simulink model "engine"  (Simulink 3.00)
settings: Solver=ode45  SolverMode=SingleTasking  StartTime=0.0  StopTime=10  RelTol=1e-3  AbsTol=1e-6

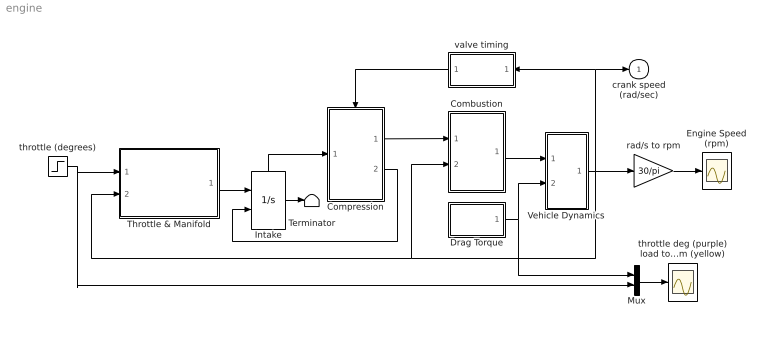
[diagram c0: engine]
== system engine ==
  Combustion : Subsystem
  Compression : Subsystem
  Drag Torque : Subsystem
  Engine Speed (rpm) : Scope
  Intake : Integrator  ExternalReset=either  InitialConditionSource=internal  InitialCondition=0  LimitOutput=off  UpperSaturationLimit=inf  LowerSaturationLimit=-inf  ShowSaturationPort=off  ShowStatePort=on  AbsoluteTolerance=auto
  Mux : Mux  Inputs=2
  Terminator : Terminator
  Throttle & Manifold : Subsystem
  Vehicle Dynamics : Subsystem
  rad/s to rpm : Gain  Gain=30/pi  SaturateOnIntegerOverflow=on
  throttle (degrees) : Step  Time=5  Before=8.973  After=11.93  SampleTime=0
  throttle deg (purple) load torque Nm (yellow) : Scope
  valve timing : Subsystem  Orientation=left
  crank speed (rad/sec) : Outport  Port=1  InitialOutput=0
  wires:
  valve timing/1(edge180) -> Compression/Trigger
  Intake/State -> Compression/1(mass(k+1))
  Intake/1 -> Terminator/1
  Throttle & Manifold/1(Mass Airflow Rate) -> Intake/1
  throttle (degrees)/1 -> Mux/2, Throttle & Manifold/1(Throttle Ang.)
  Compression/2(trigger) -> Intake/2
  Vehicle Dynamics/1(N) -> rad/s to rpm/1, crank speed (rad/sec)/1, valve timing/1(N), Combustion/2(N), Throttle & Manifold/2("Engine Speed, N")
  Compression/1(mass(k)) -> Combustion/1(Air Charge)
  rad/s to rpm/1 -> Engine Speed (rpm)/1
  Combustion/1(Torque) -> Vehicle Dynamics/1(Teng)
  Mux/1 -> throttle deg (purple) load torque Nm (yellow)/1
  Drag Torque/1(Load) -> Vehicle Dynamics/2(Tload), Mux/1

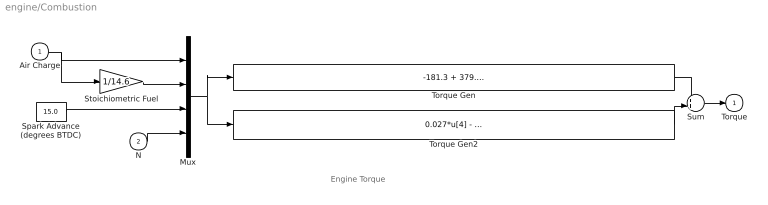
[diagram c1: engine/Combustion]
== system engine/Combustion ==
  note: Engine Torque
  Air Charge : Inport  Port=1  PortWidth=-1  SampleTime=-1  DataType=auto
  N : Inport  Port=2  PortWidth=-1  SampleTime=-1  DataType=auto
  Mux : Mux  Inputs=4
  Spark Advance (degrees BTDC) : Constant  Value=15.0
  Stoichiometric Fuel : Gain  Gain=1/14.6  SaturateOnIntegerOverflow=on
  Sum : Sum  Inputs=++  SaturateOnIntegerOverflow=on
  Torque Gen : Fcn  Expr=-181.3 + 379.36*u[1] + 21.91*u[1]/u[2] - (0.85*u[1]*u[1])/(u[2]*u[2]) + 0.26*u[3] - 0.0028*u[3]*u[3]
  Torque Gen2 : Fcn  Expr=0.027*u[4] - 0.000107*u[4]*u[4] + 0.00048*u[4]*u[3] + 2.55*u[3]*u[1] - 0.05*u[3]*u[3]*u[1]
  Torque : Outport  Port=1  InitialOutput=0
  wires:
  Sum/1 -> Torque/1
  Torque Gen/1 -> Sum/1
  Torque Gen2/1 -> Sum/2
  Mux/1 -> Torque Gen2/1, Torque Gen/1
  Air Charge/1 -> Mux/1, Stoichiometric Fuel/1
  N/1 -> Mux/4
  Spark Advance (degrees BTDC)/1 -> Mux/3
  Stoichiometric Fuel/1 -> Mux/2

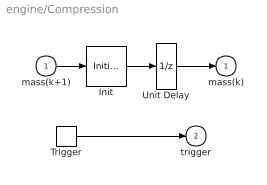
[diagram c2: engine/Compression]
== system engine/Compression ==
  mass(k+1) : Inport  Port=1  PortWidth=-1  SampleTime=-1  DataType=auto
  Trigger : TriggerPort  TriggerType=either  ShowOutputPort=on  OutputDataType=auto
  Init : InitialCondition  Value=0.152
  Unit Delay : UnitDelay  X0=0.152  SampleTime=-1
  mass(k) : Outport  Port=1  InitialOutput=0.152
  trigger : Outport  Port=2  InitialOutput=-1
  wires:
  Trigger/1 -> trigger/1
  Unit Delay/1 -> mass(k)/1
  mass(k+1)/1 -> Init/1
  Init/1 -> Unit Delay/1

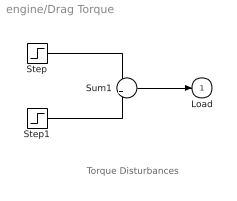
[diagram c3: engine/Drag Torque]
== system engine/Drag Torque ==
  note: Torque Disturbances
  Step : Step  Time=2  Before=25  After=20  SampleTime=0
  Step1 : Step  Time=8  Before=0  After=5  SampleTime=0
  Sum1 : Sum  Inputs=++  SaturateOnIntegerOverflow=on
  Load : Outport  Port=1  InitialOutput=0
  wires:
  Sum1/1 -> Load/1
  Step/1 -> Sum1/1
  Step1/1 -> Sum1/2

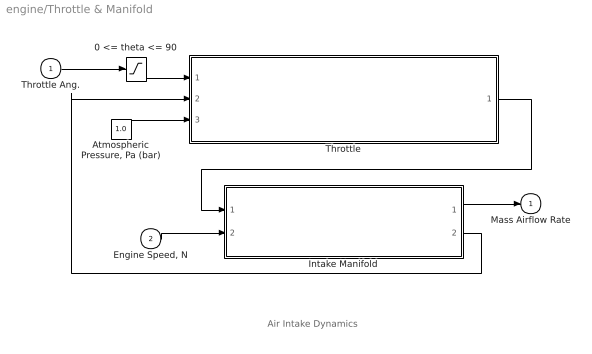
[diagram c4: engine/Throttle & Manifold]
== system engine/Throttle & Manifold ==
  note: Air Intake Dynamics
  Throttle Ang. : Inport  Port=1  PortWidth=-1  SampleTime=-1  DataType=auto
  "Engine Speed, N" : Inport  Port=2  PortWidth=-1  SampleTime=-1  DataType=auto
  0 <= theta <= 90 : Saturate  UpperLimit=90  LowerLimit=0
  "Atmospheric Pressure, Pa (bar)" : Constant  Value=1.0
  Intake Manifold : Subsystem
  Throttle : Subsystem
  Mass Airflow Rate : Outport  Port=1  InitialOutput=0
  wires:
  0 <= theta <= 90/1 -> Throttle/1("Throttle Angle, theta (deg)")
  Throttle Ang./1 -> 0 <= theta <= 90/1
  Throttle/1("Throttle  Flow, mdot  (g/s)") -> Intake Manifold/1(mdot Input  (g/s))
  "Engine Speed, N"/1 -> Intake Manifold/2(N (rad/sec))
  Intake Manifold/2("Manifold Pressure, Pm (bar)") -> Throttle/2("Manifold Pressure, Pm (bar)")
  Intake Manifold/1(mdot to  Cylinder  (g/s)) -> Mass Airflow Rate/1
  "Atmospheric Pressure, Pa (bar)"/1 -> Throttle/3("Atmospheric Pressure, Pa (bar) ")

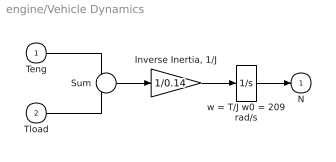
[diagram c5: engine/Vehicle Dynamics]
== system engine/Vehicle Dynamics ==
  Teng : Inport  Port=1  PortWidth=-1  SampleTime=-1  DataType=auto
  Tload : Inport  Port=2  PortWidth=-1  SampleTime=-1  DataType=auto
  "Inverse Inertia, 1/J" : Gain  Gain=1/0.14  SaturateOnIntegerOverflow=on
  Sum : Sum  Inputs=+-  SaturateOnIntegerOverflow=on
  w = T/J w0 = 209 rad/s : Integrator  ExternalReset=none  InitialConditionSource=internal  InitialCondition=209.48  LimitOutput=off  UpperSaturationLimit=inf  LowerSaturationLimit=-inf  ShowSaturationPort=off  ShowStatePort=off  AbsoluteTolerance=auto
  N : Outport  Port=1  InitialOutput=0
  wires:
  Tload/1 -> Sum/2
  Teng/1 -> Sum/1
  Sum/1 -> "Inverse Inertia, 1/J"/1
  w = T/J w0 = 209 rad/s/1 -> N/1
  "Inverse Inertia, 1/J"/1 -> w = T/J w0 = 209 rad/s/1

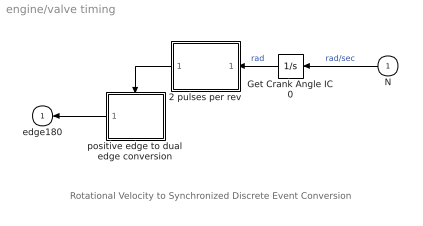
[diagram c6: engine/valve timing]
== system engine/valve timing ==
  note: Rotational Velocity to Synchronized Discrete Event Conversion
  N : Inport  Orientation=left  Port=1  PortWidth=-1  SampleTime=-1  DataType=auto
  2 pulses per rev : Subsystem  Orientation=left  mask(synchronous rotational pulse generator){Nper=2}
      mask prompts: Nper "pulses per rev (Nper)"
      mask help: A continuous angular position input (radians) is used to generate Nper timing pulses each revolution. When using a variable step-size solver, the pulses are issued at the precise instants the input crosses 2*pi/Nper. In addition, the solver is prevented from taking any steps that are so large that an entire pulse is missed.
      mask init:
      | delta = 2*pi/Nper;
  Get Crank Angle IC 0 : Integrator  Orientation=left  ExternalReset=none  InitialConditionSource=internal  InitialCondition=0  LimitOutput=off  UpperSaturationLimit=inf  LowerSaturationLimit=-inf  ShowSaturationPort=off  ShowStatePort=off  AbsoluteTolerance=auto
  positive edge to dual edge conversion : Subsystem  Orientation=left
  edge180 : Outport  Orientation=left  Port=1  InitialOutput=-1
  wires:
  N/1 -> Get Crank Angle IC 0/1  "rad/sec"
  Get Crank Angle IC 0/1 -> 2 pulses per rev/1(theta)  "rad"
  positive edge to dual edge conversion/1(trigger) -> edge180/1
  2 pulses per rev/1(trigger) -> positive edge to dual edge conversion/Trigger

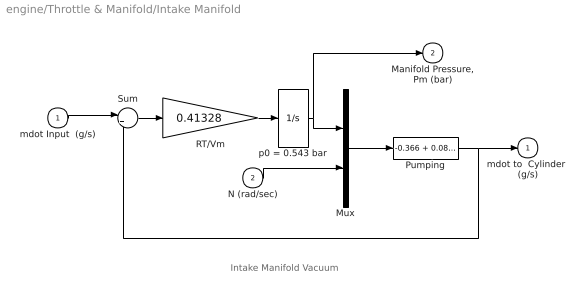
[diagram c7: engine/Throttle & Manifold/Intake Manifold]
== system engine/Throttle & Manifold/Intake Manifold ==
  note: Intake Manifold Vacuum
  mdot Input  (g/s) : Inport  Port=1  PortWidth=-1  SampleTime=-1  DataType=auto
  N (rad/sec) : Inport  Port=2  PortWidth=-1  SampleTime=-1  DataType=auto
  Mux : Mux  Inputs=2
  Pumping : Fcn  Expr=-0.366 + 0.08979*u[1]*u[2] - 0.0337*u[2]*u[1]*u[1] + 0.0001*u[1]*u[2]*u[2]
  RT/Vm : Gain  Gain=0.41328  SaturateOnIntegerOverflow=on
  Sum : Sum  Inputs=|+-  SaturateOnIntegerOverflow=on
  p0 = 0.543 bar : Integrator  ExternalReset=none  InitialConditionSource=internal  InitialCondition=.543  LimitOutput=off  UpperSaturationLimit=inf  LowerSaturationLimit=-inf  ShowSaturationPort=off  ShowStatePort=off  AbsoluteTolerance=auto
  mdot to  Cylinder  (g/s) : Outport  Port=1  InitialOutput=0
  "Manifold Pressure, Pm (bar)" : Outport  Port=2  InitialOutput=0
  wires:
  mdot Input  (g/s)/1 -> Sum/1
  RT/Vm/1 -> p0 = 0.543 bar/1
  N (rad/sec)/1 -> Mux/2
  Mux/1 -> Pumping/1
  p0 = 0.543 bar/1 -> Mux/1, "Manifold Pressure, Pm (bar)"/1
  Sum/1 -> RT/Vm/1
  Pumping/1 -> Sum/2, mdot to  Cylinder  (g/s)/1

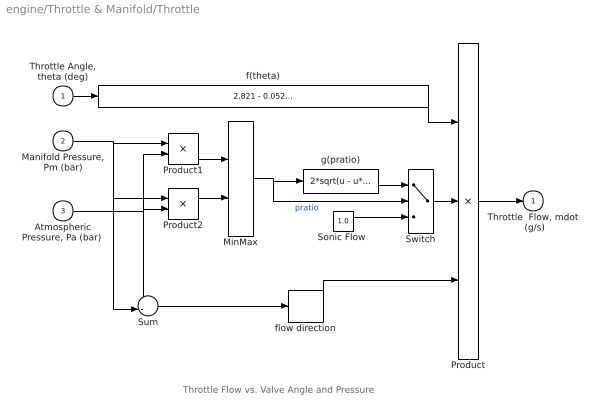
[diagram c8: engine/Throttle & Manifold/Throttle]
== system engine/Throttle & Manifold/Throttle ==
  note: Throttle Flow vs. Valve Angle and Pressure
  "Throttle Angle, theta (deg)" : Inport  Port=1  PortWidth=-1  SampleTime=-1  DataType=auto
  "Manifold Pressure, Pm (bar)" : Inport  Port=2  PortWidth=-1  SampleTime=-1  DataType=auto
  "Atmospheric Pressure, Pa (bar) " : Inport  Port=3  PortWidth=-1  SampleTime=-1  DataType=auto
  MinMax : MinMax  Function=min  Inputs=2
  Product : Product  Inputs=3  SaturateOnIntegerOverflow=on
  Product1 : Product  Inputs=*/  SaturateOnIntegerOverflow=on
  Product2 : Product  Inputs=/*  SaturateOnIntegerOverflow=on
  "Sonic Flow " : Constant  Value=1.0
  Sum : Sum  Inputs=+-|  SaturateOnIntegerOverflow=on
  Switch : Switch  Threshold=0.5
  f(theta) : Fcn  Expr=2.821 - 0.05231*u + 0.10299*u*u - 0.00063*u*u*u
  flow direction : Signum
  g(pratio) : Fcn  Expr=2*sqrt(u - u*u)
  "Throttle  Flow, mdot  (g/s)" : Outport  Port=1  InitialOutput=0
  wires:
  "Manifold Pressure, Pm (bar)"/1 -> Sum/2, Product2/1, Product1/1
  Product2/1 -> MinMax/2
  Product1/1 -> MinMax/1
  "Atmospheric Pressure, Pa (bar) "/1 -> Sum/1, Product2/2, Product1/2
  g(pratio)/1 -> Switch/1
  "Sonic Flow "/1 -> Switch/3
  Switch/1 -> Product/2
  flow direction/1 -> Product/3
  Sum/1 -> flow direction/1
  MinMax/1 -> Switch/2, g(pratio)/1  "pratio"
  "Throttle Angle, theta (deg)"/1 -> f(theta)/1
  Product/1 -> "Throttle  Flow, mdot  (g/s)"/1
  f(theta)/1 -> Product/1

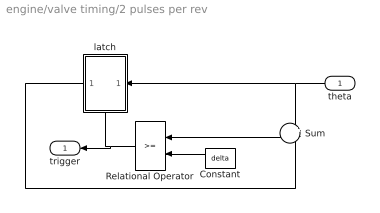
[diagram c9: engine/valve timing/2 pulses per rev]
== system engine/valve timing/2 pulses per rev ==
  theta : Inport  Orientation=left  Port=1  PortWidth=-1  SampleTime=-1  DataType=auto
  Constant : Constant  Orientation=left  Value=delta
  Relational Operator : RelationalOperator  Orientation=left  Operator=>=
  Sum : Sum  Orientation=left  Inputs=+-  SaturateOnIntegerOverflow=on
  latch : Subsystem  Orientation=left
  trigger : Outport  Orientation=left  Port=1  InitialOutput=0
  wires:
  Sum/1 -> Relational Operator/1
  theta/1 -> Sum/1, latch/1(In)
  Relational Operator/1 -> latch/Trigger, trigger/1
  Constant/1 -> Relational Operator/2
  latch/1(Out) -> Sum/2

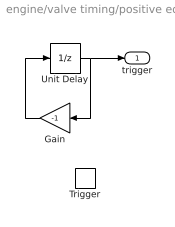
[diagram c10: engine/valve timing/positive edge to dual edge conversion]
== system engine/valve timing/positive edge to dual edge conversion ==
  Trigger : TriggerPort  TriggerType=rising  OutputDataType=auto
  Gain : Gain  Orientation=left  Gain=-1  SaturateOnIntegerOverflow=on
  Unit Delay : UnitDelay  X0=1  SampleTime=-1
  trigger : Outport  Port=1  InitialOutput=-1
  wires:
  Unit Delay/1 -> Gain/1, trigger/1
  Gain/1 -> Unit Delay/1

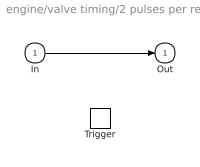
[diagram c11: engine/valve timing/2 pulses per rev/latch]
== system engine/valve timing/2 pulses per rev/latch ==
  In : Inport  Port=1  PortWidth=-1  SampleTime=-1  DataType=auto
  Trigger : TriggerPort  TriggerType=rising  OutputDataType=auto
  Out : Outport  Port=1  InitialOutput=0
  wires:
  In/1 -> Out/1
